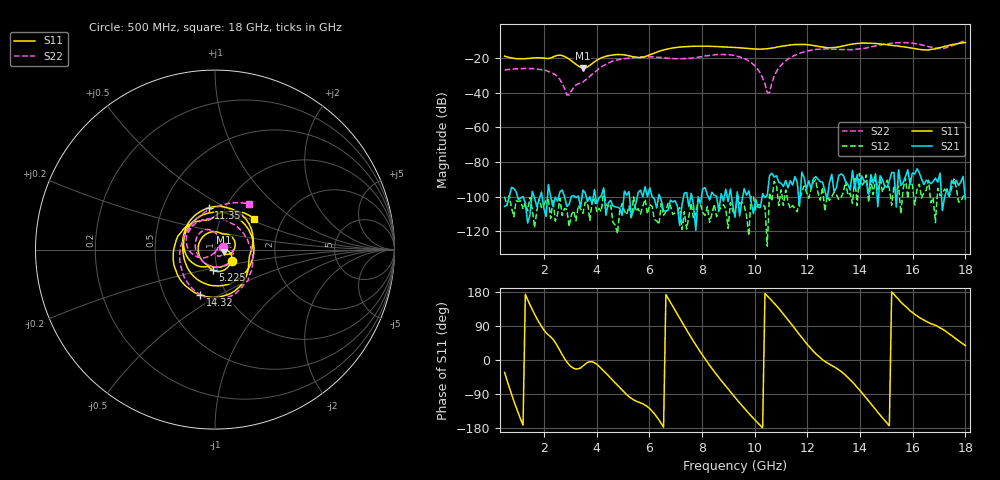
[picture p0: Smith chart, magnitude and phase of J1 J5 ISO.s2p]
!Agilent Technologies,N5230A,MY45001360,A.07.50.67
!Agilent N5230A: A.07.50.67
!Date: Tuesday, April 16, 2024 17:40:34
!Correction: S11(Full 2 Port(1,2))
!S21(Full 2 Port(1,2))
!S12(Full 2 Port(1,2))
!S22(Full 2 Port(1,2))
!S2P File: Measurements: S11, S21, S12, S22:
# Hz S  dB  R 50
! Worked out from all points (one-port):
!   201 points, 500 MHz to 18 GHz, reference 50 ohm
!   lowest |S11| = -25.8 dB at 3.475 GHz (marker M1), VSWR 1.11, Z = 55.1 - j1.55 ohm
!   |S11| at or under -10 dB: start of sweep to end of sweep
!   S11 on the Smith chart (normalised r, x): 500 MHz: 1.20, -0.15; 5.225 GHz: 0.95, -0.22; 11.35 GHz: 0.84, +0.42; 14.32 GHz: 0.75, -0.41; 18 GHz: 1.45, +0.53
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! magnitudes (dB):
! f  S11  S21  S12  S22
! 500 MHz  -19.0  -105.6  -100.0  -27.1
! 2.075 GHz  -20.3  -111.5  -101.8  -27.3
! 2.513 GHz  -18.5  -102.6  -110.1  -30.8
! 2.862 GHz  -19.8  -105.6  -107.3  -41.4
! 3.475 GHz  -25.8  -96.2  -109.6  -34.0
! 4.438 GHz  -18.7  -103.7  -105.7  -23.0
! 5.225 GHz  -18.8  -97.1  -105.5  -20.1
! 6.362 GHz  -16.2  -98.6  -116.1  -19.7
! 9.25 GHz  -13.9  -111.9  -111.0  -18.7
! 10.04 GHz  -14.9  -101.4  -107.6  -25.1
! 10.3 GHz  -14.9  -98.3  -105.2  -31.5
! 10.47 GHz  -14.7  -99.2  -128.5  -40.0
! 10.56 GHz  -14.5  -87.8  -97.7  -40.0
! 10.74 GHz  -14.1  -88.7  -91.1  -30.4
! 10.91 GHz  -13.6  -91.7  -105.2  -25.6
! 11.35 GHz  -12.5  -90.8  -107.0  -19.8
! 12.22 GHz  -12.9  -89.7  -91.4  -15.4
! 14.32 GHz  -11.6  -98.8  -103.3  -13.9
! 15.11 GHz  -12.6  -90.8  -95.4  -11.8
! 16.51 GHz  -15.4  -90.5  -96.4  -13.2
! 17.12 GHz  -13.8  -108.0  -98.0  -14.6
! 18 GHz  -11.1  -101.6  -98.9  -10.0
